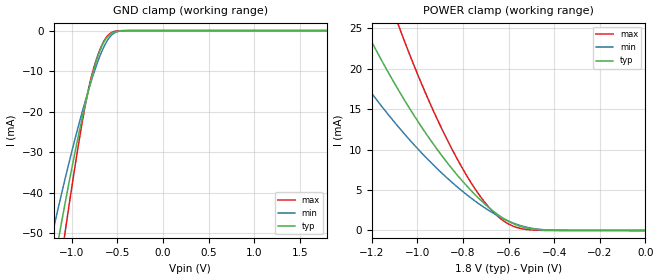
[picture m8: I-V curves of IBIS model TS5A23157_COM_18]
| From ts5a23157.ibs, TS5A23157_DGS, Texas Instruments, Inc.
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[Model]   TS5A23157_COM_18
Model_type  Terminator
| variable   typ   min   max
C_comp   16.19pF   10.75pF   18.73pF
| C_tri-state   16.19pF   10.75pF   18.73pF
[Temperature Range]   40   100   -40
| Ambient temperature   25   85   -40
[Voltage range]   1.8   1.65   1.95
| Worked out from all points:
|   GND clamp passes 1 mA (typ) near -0.58 V on its own axis
|   POWER clamp passes 1 mA (typ) near -0.59 V on its own axis
[GND Clamp]
| TS5A23157_COM_18
|   Voltage   I(typ)   I(min)   I(max)
-1.8V     -143.2mA   -115.8mA   -175.8mA
-1.205V   -59.02mA   -49.38mA   -70.87mA
-1.14V    -50.79mA   -42.96mA   -60.31mA
-1.12V    -48.31mA   -41.03mA   -57.12mA
-1.08V    -43.44mA   -37.23mA   -50.83mA
-1.06V    -41.04mA   -35.36mA   -47.73mA
-885mV    -21.51mA   -20.04mA   -22.61mA
-795mV    -12.82mA   -13.09mA   -12.3mA
-680mV    -4.313mA   -5.666mA   -4.105mA
-570mV    -793.5uA   -1.255mA   -568.8uA
-395mV    -12.13uA   -20.23uA   -2.239uA
1.8V      1.922nA    51.12nA    1.838nA
[POWER Clamp]
| TS5A23157_COM_18
|   Voltage   I(typ)   I(min)   I(max)
-1.8V     63.74mA    45.46mA    97.88mA
-1.4V     35.01mA    25.14mA    53.32mA
-1.385V   34.06mA    24.48mA    51.84mA
-1.22V    24.38mA    17.7mA     36.52mA
-1.075V   16.98mA    12.53mA    24.76mA
-955mV    11.68mA    8.812mA    16.38mA
-840mV    7.351mA    5.741mA    9.603mA
-725mV    3.808mA    3.19mA     4.237mA
-635mV    1.712mA    1.632mA    1.451mA
-570mV    720.5uA    814.8uA    422.1uA
-480mV    125.2uA    192uA      34.62uA
-16.28fV  1.922nA    2.449nA    1.997nA
